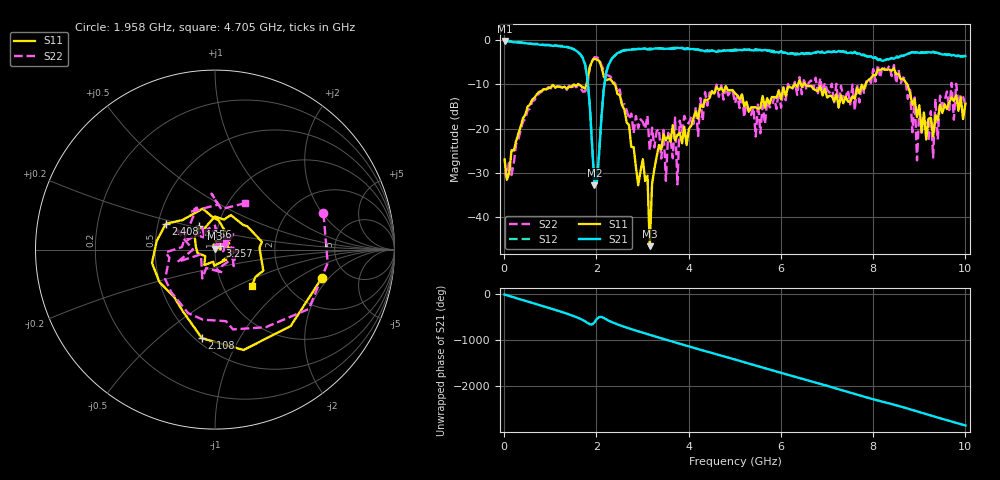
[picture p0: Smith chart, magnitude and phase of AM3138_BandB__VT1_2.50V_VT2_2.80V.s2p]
! Date/Time: Tue, Nov 13, 2018 4:39 PM
! Network Analyzer: Agilent Technologies E8364B Rev: A.07.50.67
! Sweep from 0.010 to 10.000 GHz, 201 Points, Sweep Type: LIN
! Power Supply: 2.501 V, 0.000 A
# Hz S DB R 50
!freq MagS11 AngS11 MagS21 AngS21 MagS12 AngS12 MagS22 AngS22
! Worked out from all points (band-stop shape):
!   201 points, 10 MHz to 10 GHz, reference 50 ohm
!   highest |S21| = -0.26 dB at 10 MHz (marker M1); lowest = -32.8 dB at 1.958 GHz (marker M2)
!   |S21| within 3 dB of the highest: start of sweep to 1.647 GHz; 2.43 GHz to 6.29 GHz (3.86 GHz wide, 88.5 % of centre)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
!   lowest |S11| = -46.5 dB at 3.157 GHz (marker M3), VSWR 1.01, Z = 49.8 + j0.442 ohm
!   |S11| at or under -10 dB: start of sweep to 1.603 GHz; 2.389 GHz to 6.302 GHz (3.913 GHz wide, 90 % of centre); 6.523 GHz to 7.839 GHz (1.316 GHz wide, 18.3 % of centre)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
!   |S22| runs from -32.6 to -3.9 dB; largest |S21 - S12| = 0.031
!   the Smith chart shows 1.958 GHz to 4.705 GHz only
!   S11 on the Smith chart (normalised r, x): 1.958 GHz: 3.26, -1.68; 2.108 GHz: 0.54, -0.71; 2.408 GHz: 0.55, +0.18; 3.257 GHz: 1.06, +0.05; 4.156 GHz: 0.81, +0.21; 4.705 GHz: 1.36, -0.60
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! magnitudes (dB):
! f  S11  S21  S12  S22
! 10 MHz  -27.0  -0.3  -0.2  -29.9
! 1.708 GHz  -10.7  -4.2  -4.1  -11.7
! 1.958 GHz  -4.2  -32.8  -32.8  -3.9
! 2.108 GHz  -6.0  -17.7  -17.6  -5.7
! 2.408 GHz  -10.2  -3.5  -3.5  -9.8
! 3.107 GHz  -30.6  -2.2  -2.1  -17.1
! 3.157 GHz  -46.5  -2.2  -2.0  -25.0
! 3.257 GHz  -29.1  -2.0  -1.9  -24.3
! 3.357 GHz  -23.7  -2.0  -1.9  -20.1
! 3.507 GHz  -22.6  -2.0  -2.0  -31.8
! 3.706 GHz  -22.6  -2.0  -1.8  -17.5
! 3.756 GHz  -21.5  -1.8  -1.8  -32.6
! 3.806 GHz  -20.9  -1.9  -1.8  -18.2
! 4.156 GHz  -16.1  -2.2  -2.2  -15.1
! 4.705 GHz  -10.8  -2.6  -2.5  -10.2
! 5.005 GHz  -12.1  -2.4  -2.2  -14.3
! 6.703 GHz  -11.0  -3.0  -2.9  -11.1
! 8.352 GHz  -6.7  -4.4  -4.4  -5.8
! 8.901 GHz  -13.4  -2.9  -2.9  -13.0
! 8.951 GHz  -17.4  -2.8  -2.7  -27.2
! 9.001 GHz  -14.8  -3.0  -2.9  -15.6
! 10 GHz  -14.4  -3.6  -3.5  -14.6
